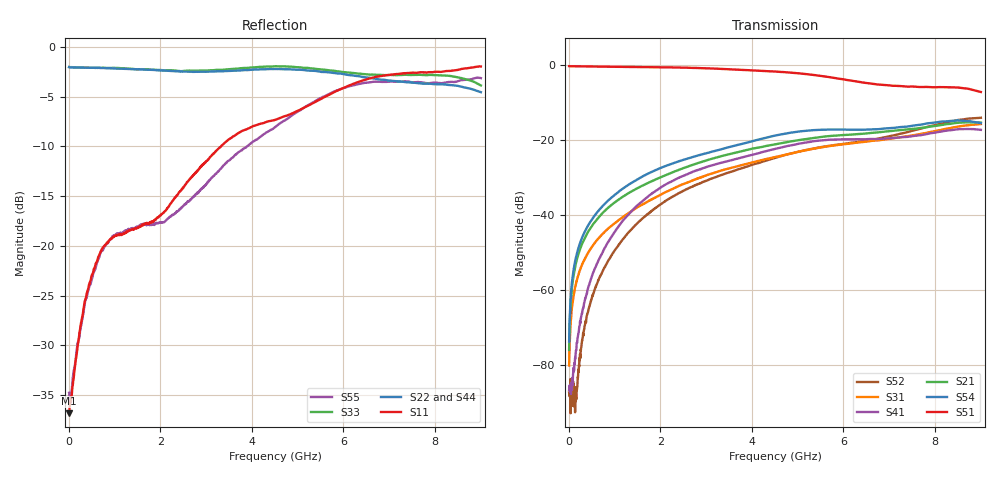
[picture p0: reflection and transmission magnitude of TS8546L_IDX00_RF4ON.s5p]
# GHz S DB R 50
! CMT, SN0916, 25263762, 26.7.0
! Date: 16.07.2026 08:37:23
! Data: Format
! Freq S1.1:dB/Ang S1.2:dB/Ang S1.3:dB/Ang S1.4:dB/Ang S1.5:dB/Ang
!  S2.1:dB/Ang S2.2:dB/Ang S2.3:dB/Ang S2.4:dB/Ang S2.5:dB/Ang
!  S3.1:dB/Ang S3.2:dB/Ang S3.3:dB/Ang S3.4:dB/Ang S3.5:dB/Ang
!  S4.1:dB/Ang S4.2:dB/Ang S4.3:dB/Ang S4.4:dB/Ang S4.5:dB/Ang
!  S5.1:dB/Ang S5.2:dB/Ang S5.3:dB/Ang S5.4:dB/Ang S5.5:dB/Ang
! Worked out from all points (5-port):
!   2001 points, 10 MHz to 9 GHz, reference 50 ohm
!   strongest paths, dB at 10 MHz, 2.257 GHz, 4.505 GHz, 6.753 GHz, 9 GHz:
!     S51: -0.2, -0.5, -1.6, -5.1, -7.1
!     S54: -73.7, -26.2, -18.7, -17.0, -15.4
!     S21: -75.9, -28.5, -21.0, -17.9, -15.3
!     S41: -86.6, -30.9, -22.2, -19.6, -17.2
!     S31: -80.1, -33.0, -24.4, -20.0, -15.6
!     S52: -87.3, -35.1, -24.7, -19.5, -14.0
!   lowest |S11| = -36.8 dB at 10 MHz (marker M1), VSWR 1.03, Z = 51.5 - j0.0611 ohm
!   |S11| at or under -10 dB: start of sweep to 3.329 GHz
